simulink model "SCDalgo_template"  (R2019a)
settings: configuration reference "configurationSettings" (kept in a data dictionary, not in this file)
undefined symbols (not defined in the file or in its folder): ProductionState, QualityTag, SCDalgo_template_fp, SCDalgo_template_tp, SCDsignal_example_1, single_scalar, Value

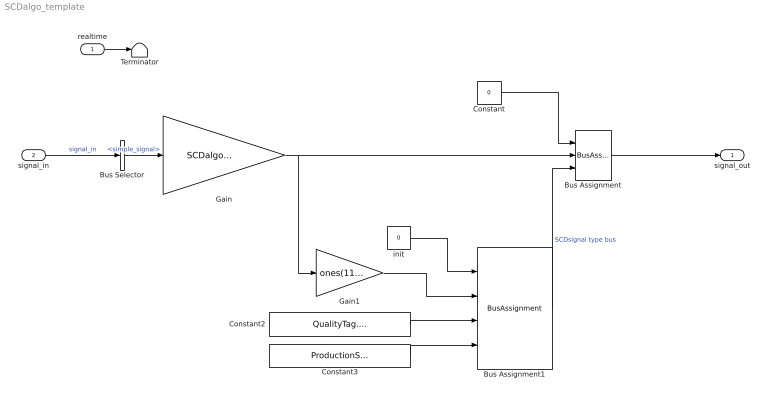
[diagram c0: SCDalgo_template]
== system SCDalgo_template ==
  realtime : Inport  OutDataTypeStr=single  PortDimensions=1  SampleTime=SCDalgo_template_fp.timing.dt  Interpolate=off
  signal_in : Inport  Port=2  OutDataTypeStr=Bus: SCDalgo_template_inBus  PortDimensions=1  SampleTime=SCDalgo_template_fp.timing.dt  Interpolate=off
  Bus Assignment : BusAssignment  AssignedSignals=single_scalar,SCDsignal_example_1
  Bus Assignment1 : BusAssignment  AssignedSignals=Value,QualityTag,ProductionState
  Bus Selector : BusSelector  OutputSignals=simple_signal
  Constant : Constant  Value=0  OutDataTypeStr=Bus: SCDalgo_template_outBus
  Constant2 : Constant  Value=QualityTag.GOOD  OutDataTypeStr=Enum: QualityTag
  Constant3 : Constant  Value=ProductionState.RUNNING  OutDataTypeStr=Enum: ProductionState
  Gain : Gain  Gain=SCDalgo_template_tp.gain
  Gain1 : Gain  Gain=ones(11,1)
  Terminator : Terminator
  init : Constant  Value=0  OutDataTypeStr=Bus: SCDBus_single_11_Vector
  signal_out : Outport  OutDataTypeStr=Bus: SCDalgo_template_outBus
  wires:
  signal_in/1 -> Bus Selector/1  "signal_in"
  Bus Selector/1 -> Gain/1  "<simple_signal>"
  Constant/1 -> Bus Assignment/1
  realtime/1 -> Terminator/1
  Bus Assignment/1 -> signal_out/1
  init/1 -> Bus Assignment1/1
  Bus Assignment1/1 -> Bus Assignment/3  "SCDsignal type bus"
  Constant2/1 -> Bus Assignment1/3
  Constant3/1 -> Bus Assignment1/4
  Gain/1 -> Gain1/1, Bus Assignment/2
  Gain1/1 -> Bus Assignment1/2
